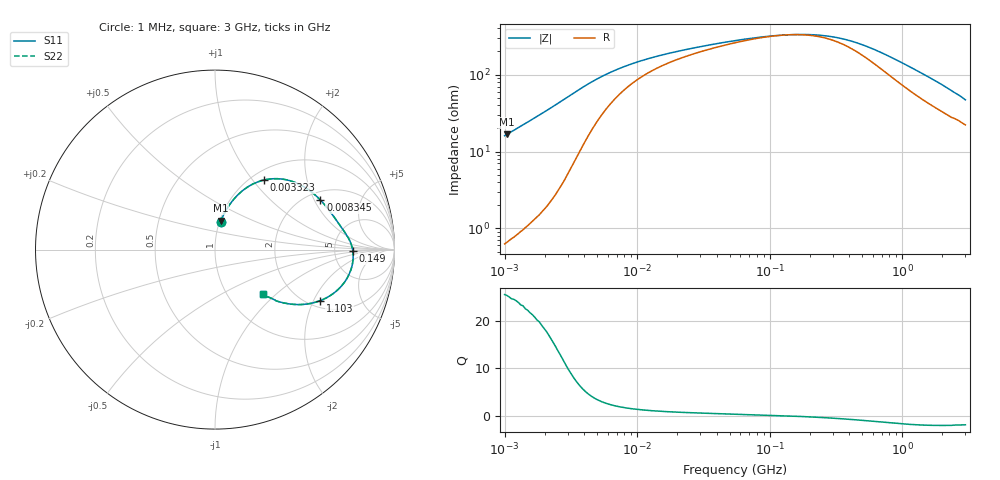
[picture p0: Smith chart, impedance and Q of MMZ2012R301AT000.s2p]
! S-parameter Generated by TDK Corporation
! Copyright(C) 2016 TDK Corporation.
! All Rights Reserved.
! TDK P/N: MMZ2012R301AT000 (Chip Beads)
! Property: |Z|=300¶ at 100MHz
! Size(LxWxT): 2x1.25x0.85mm, 0.079x0.049x0.033inches
! Model Type: s2p (Touchstone File Format Version 1.0)
! Frequency: DC=Yes Start=1MHz Stop=3000MHz 202points Log-sweep
! Note: This model was converted from impedance.
! Model Generated on May. 16, 2016
! Hash(MD5):
! Port Assignments:
!  1 ---@@@--- 2
! Applicable Conditions:
!  Temperature = 25 degC
!  DC Bias Current = 0 A
!  Small Signal Operation
! Terms and conditions regarding TDK Simulation Models
! (1)This simulation model is being provided solely for informational purposes. Please refer to the specifications of the products in terms of detailed characteristics of such products.
! (2)In no event shall TDK Corporation of any of its subsidiaries be liable for any loss or damage arising, directly or indirectly,
!  From any information contained in this simulation model, including, but not limited to loss or damages arising from any inaccuracies, omissions or errors in connection with such information.
! (3)Any and all copyrights on this simulation model are owned by TDK Corporation.
!  Duplication or redistribution of this simulation model without prior written permission from TDK Corporation is prohibited.
! (4)This simulation model is subject to any modification or change without any prior notice.
! (5)Neither TDK Corporation nor any of its subsidiaries shall make any warranty, express or implied,
!  Including but not limited to the correctness, implied warranties of merchantability and fitness for a particular purpose with respect to this simulation models.
! (6)The use of this simulation model shall be deemed to have consented to the terms and conditions hereof.
# MHz S MA R 50
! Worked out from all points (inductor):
!   201 points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, 1 MHz to 3 GHz, reference 50 ohm
!   read as one part in series: L = 2.56 uH near 1.041 MHz
!   highest Q = 25.3 at 1.041 MHz (marker M1), where L = 2.55 uH
!   self-resonance near 136 MHz
!   S11 on the Smith chart (normalised r, x): 1 MHz: 1.01, +0.32; 3.323 MHz: 1.14, +1.14; 8.345 MHz: 2.35, +2.24; 149 MHz: 7.62, -0.30; 1.103 GHz: 2.29, -2.26; 3 GHz: 1.44, -0.83
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1  0.1576 78.7  0.9814 -9.1  0.9814 -9.1  0.1576 78.7
1.040844  0.1638 78.3  0.98 -9.4  0.98 -9.4  0.1638 78.3
1.4923  0.2321 74.0  0.9623 -13.4  0.9623 -13.4  0.2321 74.0
2.055611  0.3147 68.5  0.9318 -18.3  0.9318 -18.3  0.3147 68.5
2.613693  0.3916 62.6  0.8906 -23.0  0.8906 -23.0  0.3916 62.6
3.32329  0.4747 54.8  0.8234 -28.1  0.8234 -28.1  0.4747 54.8
3.900413  0.5251 48.8  0.7642 -31.1  0.7642 -31.1  0.5251 48.8
5.592179  0.6039 35.8  0.6207 -34.7  0.6207 -34.7  0.6039 35.8
8.345207  0.6489 25.2  0.4963 -33.8  0.4963 -33.8  0.6489 25.2
14.61624  0.6852 15.9  0.3895 -28.9  0.3895 -28.9  0.6852 15.9
54.77226  0.7436 5.3  0.2687 -14.9  0.2687 -14.9  0.7436 5.3
99.84923  0.761 1.9  0.2407 -5.9  0.2407 -5.9  0.761 1.9
149.005  0.7682 -0.6  0.2319 2.0  0.2319 2.0  0.7682 -0.6
213.6344  0.7711 -3.2  0.234 10.5  0.234 10.5  0.7711 -3.2
294.2768  0.7699 -5.9  0.2474 18.8  0.2474 18.8  0.7699 -5.9
389.4533  0.7641 -8.9  0.2723 25.8  0.2723 25.8  0.7641 -8.9
581.181  0.743 -14.4  0.3355 33.4  0.3355 33.4  0.743 -14.4
800.5644  0.7076 -19.8  0.411 35.6  0.411 35.6  0.7076 -19.8
1102.76  0.6526 -25.8  0.5009 34.6  0.5009 34.6  0.6526 -25.8
1782.824  0.5317 -35.0  0.6417 28.4  0.6417 28.4  0.5317 -35.0
2266.846  0.4578 -39.3  0.7076 24.2  0.7076 24.2  0.4578 -39.3
3000  0.3642 -43.1  0.7751 18.7  0.7751 18.7  0.3642 -43.1
